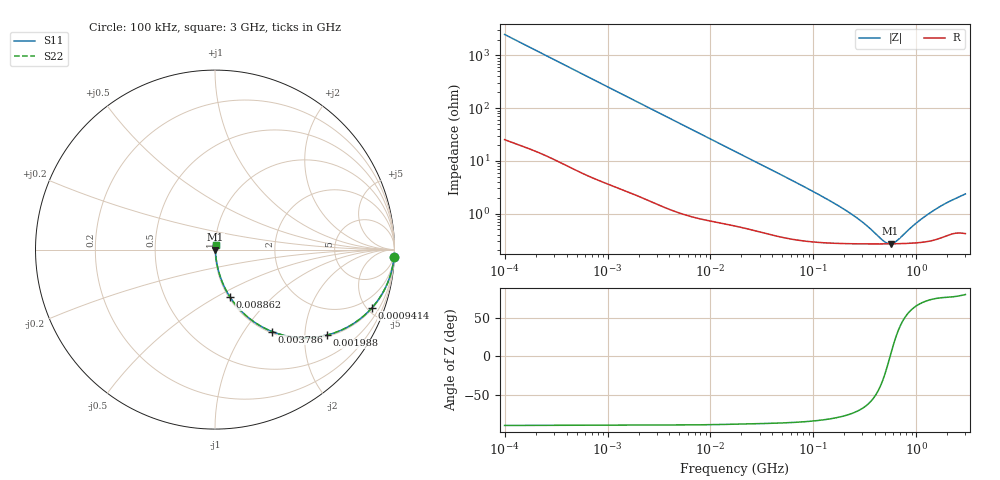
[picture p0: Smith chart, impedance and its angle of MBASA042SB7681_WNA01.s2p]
! MBASA042SB7681_WNA01  S-PARAMETER MODEL  ( Standard Model )
! Model Generated by TAIYO YUDEN Corporation (https://www.yuden.co.jp/en/)
! Version 1.0
! TAIYO YUDEN Control No. 250312
! Copyright(c) 2025 TAIYO YUDEN CO.,LTD. All Rights Reserved.
! Product Description (link to TY-COMPAS)
! https://ds.yuden.co.jp/TYCOMPAS/or/detail?pn=MBASA042SB7681KWNA01&u=M
! Products Name : Multilayer Ceramic Capacitors
! Characteristics :
!  Capacitance : 680 [pF] , Rated Voltage : 4 [V] , TCC : X7R
!  Case Size : 0.4 x 0.2 / 0.016 x 0.008 [mm/inch] , Thickness : 0.2 / 0.008 [mm/inch]
!  (Conditions: Temperature = 25 [degC] , DC Bias Voltage = 0 [V])
! External Node Assignments :
!  1  o---| |---o  2
! GND o---------o GND
! Frequency Range : 100kHz  -  3GHz  [ 401 STEP ]
# MHZ S RI R 50
! Freq[MHz].  S11 Real  S11 Imag  S21 Real  S21 Imag  S12 Real  S12 Imag  S22 Real  S22 Imag
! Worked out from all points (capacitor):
!   401 points, 100 kHz to 3 GHz, reference 50 ohm
!   read as one part in series: C = 636 pF near 105.3 kHz
!   lowest |Z| = 267 mohm at 561.8 MHz (marker M1)
!   series resonance near 557.2 MHz, so ESL is about 130 pH
!   S11 on the Smith chart (normalised r, x): 100 kHz: 2, -50; 941.4 kHz: 1.08, -5.40; 1.988 MHz: 1.04, -2.57; 3.786 MHz: 1.03, -1.36; 8.862 MHz: 1.02, -0.58; 3 GHz: 1.01, +0.05
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0.1  0.998 -0.0399  0.002 0.0399  0.002 0.0399  0.998 -0.0399
0.259498  0.9882 -0.1018  0.0118 0.1018  0.0118 0.1018  0.9882 -0.1018
0.562235  0.9505 -0.2105  0.0495 0.2105  0.0495 0.2105  0.9505 -0.2105
0.941399  0.8759 -0.3227  0.1241 0.3227  0.1241 0.3227  0.8759 -0.3227
1.350433  0.7773 -0.4084  0.2227 0.4084  0.2227 0.4084  0.7773 -0.4084
1.987766  0.6217 -0.4767  0.3783 0.4767  0.3783 0.4767  0.6217 -0.4767
3.161081  0.3998 -0.481  0.6002 0.481  0.6002 0.481  0.3998 -0.481
3.78604  0.3193 -0.4571  0.6807 0.4571  0.6807 0.4571  0.3193 -0.4571
5.718342  0.1745 -0.3692  0.8255 0.3692  0.8255 0.3692  0.1745 -0.3692
8.862326  0.0845 -0.2656  0.9155 0.2656  0.9155 0.2656  0.0845 -0.2656
17.7727  0.0265 -0.1423  0.9735 0.1423  0.9735 0.1423  0.0265 -0.1423
37.52708  0.00889 -0.0695  0.9911 0.0695  0.9911 0.0695  0.00889 -0.0695
97.38194  0.00361 -0.0265  0.9964 0.0265  0.9964 0.0265  0.00361 -0.0265
233.9019  0.00276 -0.00942  0.9972 0.00942  0.9972 0.00942  0.00276 -0.00942
318.6746  0.00269 -0.00565  0.9973 0.00565  0.9973 0.00565  0.00269 -0.00565
481.3181  0.00266 -0.00141  0.9973 0.00141  0.9973 0.00141  0.00266 -0.00141
547.5153  0.00266 -0.000168  0.9973 0.000168  0.9973 0.000168  0.00266 -0.000168
561.8095  0.00267 8.01e-05  0.9973 -8.01e-05  0.9973 -8.01e-05  0.00267 8.01e-05
639.0768  0.00268 0.00132  0.9973 -0.00132  0.9973 -0.00132  0.00268 0.00132
990.4458  0.00281 0.00587  0.9972 -0.00587  0.9972 -0.00587  0.00281 0.00587
1420.79  0.00317 0.0104  0.9968 -0.0104  0.9968 -0.0104  0.00317 0.0104
3000  0.00469 0.023  0.9953 -0.023  0.9953 -0.023  0.00469 0.023
